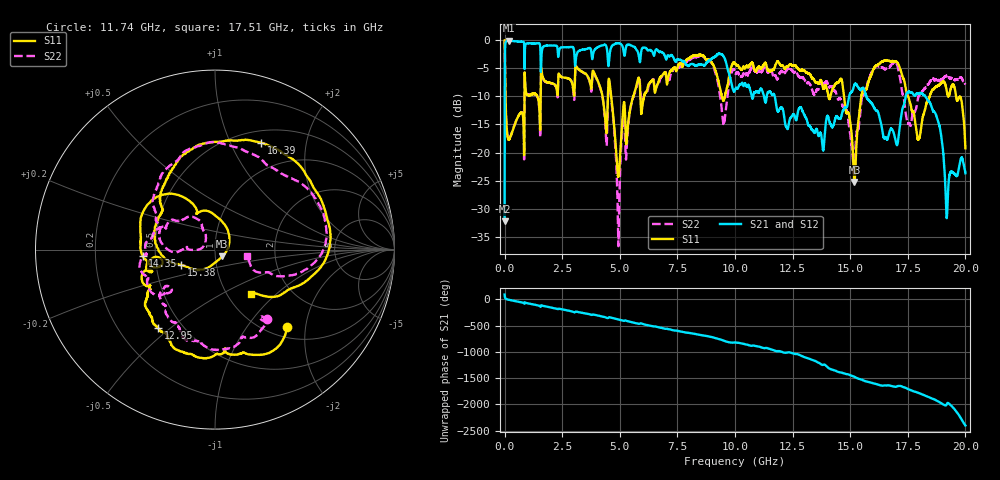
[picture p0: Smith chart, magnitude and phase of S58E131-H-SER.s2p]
!{S58E131}
!Johanson Technology Inc.
!www.johansontechnology.com
!Test Board Conditions:
!Substrate Type  RO4350B
!Substrate Thickness  60 mil
!Substrate Dk  3.66
!TL Type: GCPW
!TL Trace Width  115 mil
!TL Gap  52 mil
!Electrode orientation  Horizontal
!DUT TOPOLOGY	SERIES
!Mounting Pad LxW  55x428 mil! Created Wed Apr 14 11:08:53 2021
# mhz S ma R 50
! 2 Port Network Data from SP1.SP block
! freq  magS11  angS11  magS21  angS21  magS12  angS12  magS22  angS22
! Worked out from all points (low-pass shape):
!   20001 points, 300 kHz to 20 GHz, reference 50 ohm
!   highest |S21| = -0.08 dB at 202.3 MHz (marker M1); lowest = -32.2 dB at 300 kHz (marker M2)
!   |S21| within 3 dB of the highest: 1.596 GHz to 3.035 GHz (1.439 GHz wide, 62.1 % of centre); 4.546 GHz to 5.838 GHz (1.292 GHz wide, 24.9 % of centre)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
!   lowest |S11| = -25.3 dB at 15.19 GHz (marker M3), VSWR 1.12, Z = 53.9 - j4.12 ohm
!   |S11| at or under -10 dB: 37.96 MHz to 862.8 MHz (824.8 MHz wide, 183 % of centre); 4.626 GHz to 5.584 GHz (958.7 MHz wide, 18.8 % of centre); 17.51 GHz to 18.45 GHz (930.5 MHz wide, 5.18 % of centre)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
!   |S22| runs from -36.7 to 0.0 dB; largest |S21 - S12| = 0.0086
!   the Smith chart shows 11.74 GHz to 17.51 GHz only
!   S11 on the Smith chart (normalised r, x): 11.74 GHz: 1.19, -1.58; 12.95 GHz: 0.37, -0.45; 14.35 GHz: 0.42, -0.03; 15.38 GHz: 0.67, -0.12; 16.39 GHz: 0.64, +1.31; 17.51 GHz: 1.29, -0.70
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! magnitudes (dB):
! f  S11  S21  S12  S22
! 300 kHz  0.0  -32.2  -32.2  0.0
! 202.3 MHz  -17.6  -0.1  -0.1  -17.5
! 3.334 GHz  -5.5  -1.7  -1.7  -5.5
! 4.586 GHz  -8.5  -1.8  -1.8  -8.7
! 4.935 GHz  -24.3  -0.5  -0.5  -36.3
! 5.757 GHz  -7.4  -1.9  -1.8  -7.8
! 6.667 GHz  -7.6  -1.9  -1.9  -8.0
! 8.589 GHz  -2.7  -4.4  -4.4  -2.8
! 9.515 GHz  -10.6  -2.9  -3.0  -14.9
! 10 GHz  -4.1  -8.8  -8.9  -5.6
! 11.74 GHz  -4.6  -10.3  -10.3  -6.3
! 12.95 GHz  -5.4  -12.8  -12.7  -6.7
! 13.33 GHz  -6.7  -15.9  -15.8  -8.7
! 14.35 GHz  -7.9  -14.1  -14.1  -9.1
! 15.19 GHz  -25.3  -7.9  -7.9  -22.6
! 15.38 GHz  -13.7  -8.5  -8.5  -15.2
! 16.39 GHz  -3.8  -16.1  -16.0  -4.9
! 16.67 GHz  -3.6  -17.0  -16.8  -4.9
! 17.51 GHz  -10.0  -9.2  -9.2  -14.8
! 18.75 GHz  -8.2  -13.6  -13.7  -7.1
! 19.2 GHz  -9.1  -31.5  -31.4  -6.3
! 20 GHz  -19.3  -23.7  -23.5  -7.9
